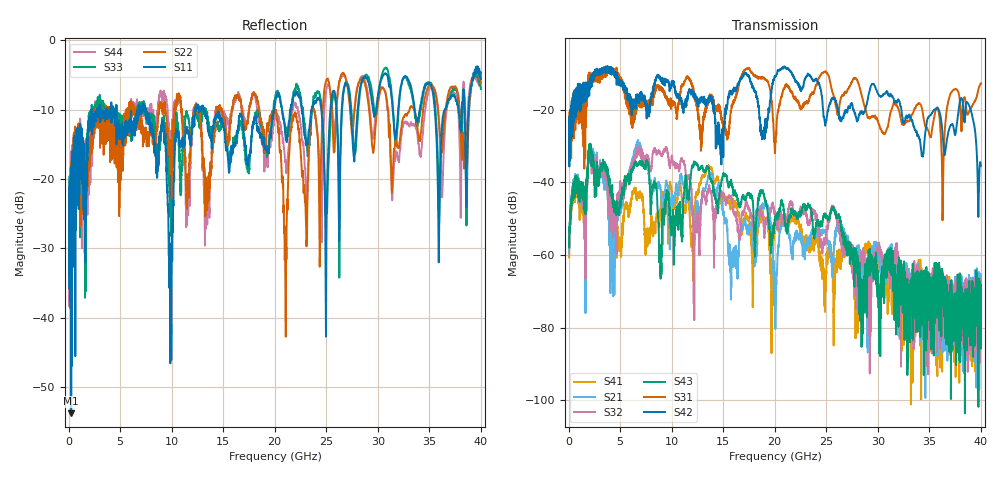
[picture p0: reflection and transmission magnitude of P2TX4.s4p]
!Agilent Technologies,N5245A,MY49151084,A.09.20.08
!Agilent N5245A: A.09.20.08
!Date: Thursday, March 01, 2012 14:21:26
!Correction: S11(Full 4 Port(1,2,3,4))
!S12(Full 4 Port(1,2,3,4))
!S13(Full 4 Port(1,2,3,4))
!S14(Full 4 Port(1,2,3,4))
!S21(Full 4 Port(1,2,3,4))
!S22(Full 4 Port(1,2,3,4))
!S23(Full 4 Port(1,2,3,4))
!S24(Full 4 Port(1,2,3,4))
!S31(Full 4 Port(1,2,3,4))
!S32(Full 4 Port(1,2,3,4))
!S33(Full 4 Port(1,2,3,4))
!S34(Full 4 Port(1,2,3,4))
!S41(Full 4 Port(1,2,3,4))
!S42(Full 4 Port(1,2,3,4))
!S43(Full 4 Port(1,2,3,4))
!S44(Full 4 Port(1,2,3,4))
!S4P File: Measurements: <S11,S12,S13,S14>,
!<S21,S22,S23,S24>,
!<S31,S32,S33,S34>,
!<S41,S42,S43,S44>:
# Hz S  dB  R 50
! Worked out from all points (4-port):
!   3996 points, 50 MHz to 40 GHz, reference 50 ohm
!   strongest paths, dB at 50 MHz, 10.04 GHz, 20.03 GHz, 30.02 GHz, 40 GHz:
!     S42: -24.5, -12.8, -10.8, -15.5, -35.3
!     S31: -24.8, -18.8, -31.1, -23.1, -12.7
!     S43: -55.2, -53.3, -49.8, -70.5, -69.9
!     S32: -56.6, -33.5, -48.2, -58.0, -77.3
!     S21: -59.4, -43.6, -70.2, -57.8, -73.8
!     S41: -60.7, -44.3, -51.1, -61.5, -80.3
!   lowest |S11| = -53.8 dB at 250 MHz (marker M1), VSWR 1.00, Z = 50.1 + j0.183 ohm
!   |S11| at or under -10 dB: start of sweep to 2.23 GHz; 7.465 GHz to 12.29 GHz (4.827 GHz wide, 48.9 % of centre); 13.13 GHz to 19.9 GHz (6.772 GHz wide, 41 % of centre)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
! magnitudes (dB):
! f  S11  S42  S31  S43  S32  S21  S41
! 50 MHz  -24.8  -24.5  -24.8  -55.2  -56.6  -59.4  -60.7
! 250 MHz  -53.8  -27.0  -33.4  -45.7  -46.0  -44.9  -46.4
! 9.4 GHz  -15.0  -11.8  -16.3  -46.7  -30.5  -40.9  -44.4
! 12.26 GHz  -10.7  -16.8  -16.0  -34.8  -51.1  -51.7  -47.0
! 21.04 GHz  -13.7  -8.4  -13.2  -51.3  -50.0  -51.3  -49.7
! 36.29 GHz  -11.1  -27.0  -48.4  -69.4  -74.0  -68.2  -79.0
! 40 GHz  -5.6  -35.3  -12.7  -69.9  -77.3  -73.8  -80.3
